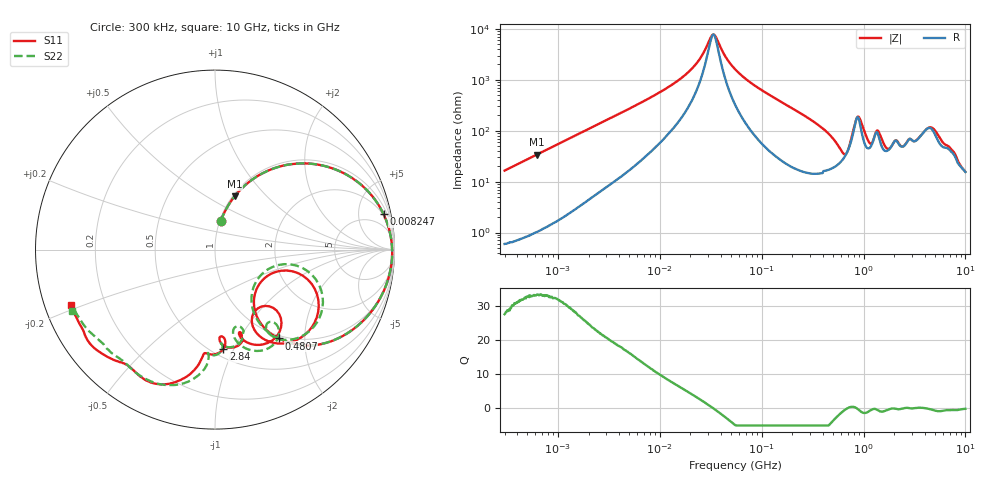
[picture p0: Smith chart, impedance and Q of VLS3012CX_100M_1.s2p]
! S-Parameter Data Generated by TDK Corporation
! Copyright(C) 2019 TDK Corporation.
! All Rights Reserved.
! TDK P/N: VLS3012CX-100M-1 (Inductor)
! Property: L=10uH at 1MHz
! Size(LxWxT): 3x3x1.2mm
! Model Type: s2p (Touchstone File Format Version 1.0)
! Frequency: DC=Yes Start=0.3MHz Stop=10000MHz 802points Log-sweep
! Model Generated on Sep. 23, 2019
! Port Assignments:
!  1 ---@@@--- 2
! Applicable Conditions:
!  Temperature = 25 degC
!  DC Bias Current = 0 A
!  Small Signal Operation
! Terms and conditions regarding TDK Simulation Models
! (1)This simulation model is being provided solely for informational purposes. Please refer to the specifications of the products in terms of detailed characteristics of such products.
! (2)In no event shall TDK Corporation of any of its subsidiaries be liable for any loss or damage arising, directly or indirectly,
!  From any information contained in this simulation model, including, but not limited to loss or damages arising from any inaccuracies, omissions or errors in connection with such information.
! (3)Any and all copyrights on this simulation model are owned by TDK Corporation.
!  Duplication or redistribution of this simulation model without prior written permission from TDK Corporation is prohibited.
! (4)This simulation model is subject to any modification or change without any prior notice.
! (5)Neither TDK Corporation nor any of its subsidiaries shall make any warranty, express or implied,
!  Including but not limited to the correctness, implied warranties of merchantability and fitness for a particular purpose with respect to this simulation models.
! (6)The use of this simulation model shall be deemed to have consented to the terms and conditions hereof.
# Hz S MA R 50
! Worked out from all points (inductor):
!   801 points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, 300 kHz to 10 GHz, reference 50 ohm
!   read as one part in series: L = 8.71 uH near 318.3 kHz
!   highest Q = 33.1 at 619.1 kHz (marker M1), where L = 8.69 uH
!   self-resonance near 33.58 MHz
!   S11 on the Smith chart (normalised r, x): 300 kHz: 1.01, +0.33; 8.247 MHz: 1.85, +9.25; 480.7 MHz: 0.95, -1.50; 2.84 GHz: 0.57, -0.91; 10 GHz: 0.08, -0.18
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300000  0.1612 78.6  0.981 -9.3  0.9812 -9.3  0.161 78.6
619123  0.3173 69.7  0.9388 -18.5  0.9389 -18.5  0.3172 69.7
1713600  0.6674 46.0  0.7199 -41.9  0.7199 -41.9  0.6672 46.0
8246826  0.9597 11.9  0.2102 -73.2  0.2103 -73.2  0.9597 11.9
9671944  0.967 9.9  0.177 -74.5  0.177 -74.5  0.967 9.9
2.126252e7  0.9846 2.5  0.05606 -73.0  0.05608 -73.0  0.9845 2.5
3.337006e7  0.9873 -0.9  0.01273 -4.1  0.01275 -4.2  0.9871 -0.9
5.477226e7  0.986 -4.9  0.06084 73.5  0.06085 73.5  0.9858 -4.9
1.563148e8  0.949 -19.0  0.2562 67.0  0.2562 67.0  0.9488 -18.9
3.126428e8  0.8259 -38.1  0.4972 46.9  0.4972 46.9  0.8254 -38.1
4.807079e8  0.6086 -54.4  0.679 23.9  0.679 23.9  0.6059 -54.7
6.407886e8  0.348 -51.2  0.7429 -1.9  0.7429 -1.9  0.3322 -52.2
7.612374e8  0.4176 -16.2  0.5935 -24.4  0.5935 -24.4  0.3957 -11.8
8.758105e8  0.6714 -31.1  0.3337 -12.6  0.3337 -12.6  0.6695 -26.0
9.903836e8  0.6523 -53.2  0.4724 8.2  0.4724 8.2  0.6717 -47.4
1.133369e9  0.4781 -63.8  0.6082 -5.4  0.6083 -5.4  0.5393 -57.3
1.260284e9  0.4208 -48.2  0.551 -19.8  0.551 -19.8  0.5234 -51.0
1.481453e9  0.5929 -62.8  0.5312 -8.8  0.5312 -8.8  0.6006 -69.5
1.767019e9  0.4888 -74.1  0.6159 -25.5  0.6159 -25.5  0.4587 -77.1
2.840323e9  0.556 -85.3  0.4548 -53.1  0.4549 -53.1  0.581 -88.1
5.040844e9  0.8144 -113.2  0.2455 -59.3  0.2455 -59.3  0.8066 -111.2
1e10  0.8594 -159.0  0.2133 -91.2  0.2133 -91.2  0.8701 -156.8
